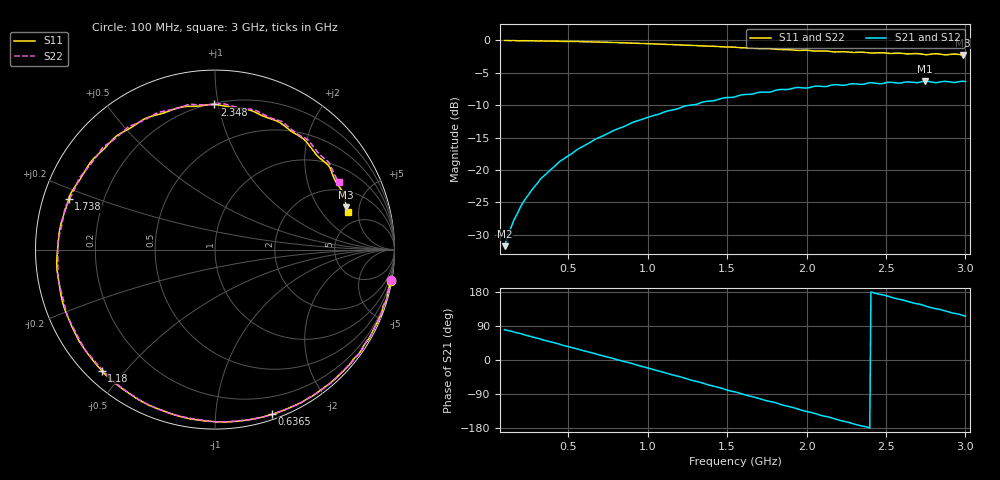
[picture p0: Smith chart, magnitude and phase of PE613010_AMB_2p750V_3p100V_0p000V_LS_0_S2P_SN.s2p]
!Agilent Technologies,N5230A,MY45001685,A.07.50.67
!Agilent N5230A: A.07.50.67
!Date: Monday, March 06, 2017 15:09:25
!Correction: S11(Full 2 Port(1,2))
!S21(Full 2 Port(1,2))
!S12(Full 2 Port(1,2))
!S22(Full 2 Port(1,2))
!S2P File: Measurements: S11, S21, S12, S22:
# Hz S  dB  R 50
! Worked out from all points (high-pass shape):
!   401 points, 100 MHz to 3 GHz, reference 50 ohm
!   highest |S21| = -6.31 dB at 2.746 GHz (marker M1); lowest = -31.7 dB at 100 MHz (marker M2)
!   |S21| within 3 dB of the highest: 1.417 GHz to end of sweep
!   lowest |S11| = -2.3 dB at 2.986 GHz (marker M3), VSWR 7.64, Z = 160 + j184 ohm
!   |S11| at or under -10 dB: nowhere
!   |S22| runs from -2.1 to 0.0 dB; largest |S21 - S12| = 0.0023
!   S11 on the Smith chart (normalised r, x): 100 MHz: 0, -11; 636.5 MHz: 0.04, -1.40; 1.18 GHz: 0.05, -0.43; 1.738 GHz: 0.08, +0.17; 2.348 GHz: 0.21, +0.97; 3 GHz: 3.67, +3.77
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1e8  -0.04 -10.2  -31.74 80.1  -31.77 80.1  -0.03 -9.9
2.015e8  -0.06 -20.9  -25.61 69.5  -25.63 69.5  -0.06 -20.2
2.8125e8  -0.08 -30.3  -22.77 60.0  -22.76 60.1  -0.09 -29.2
4.8425e8  -0.18 -53.7  -18.08 36.9  -18.09 37.0  -0.16 -52.1
5.8575e8  -0.23 -64.7  -16.46 25.6  -16.47 25.6  -0.21 -63.5
6.365e8  -0.25 -70.9  -15.78 20.3  -15.78 20.2  -0.25 -68.0
8.4675e8  -0.40 -94.5  -13.35 -3.3  -13.36 -3.4  -0.37 -91.3
1.0715e9  -0.59 -120.2  -11.38 -29.1  -11.37 -29.2  -0.57 -117.0
1.18025e9  -0.69 -133.1  -10.62 -41.8  -10.62 -41.8  -0.68 -129.3
1.376e9  -0.91 -156.8  -9.40 -64.9  -9.40 -65.0  -0.90 -152.1
1.55e9  -1.08 -176.3  -8.72 -84.1  -8.71 -84.1  -1.05 -170.9
1.7385e9  -1.28 161.0  -8.00 -106.5  -8.00 -106.6  -1.26 166.3
1.898e9  -1.46 142.8  -7.51 -123.5  -7.51 -123.6  -1.42 150.3
1.9705e9  -1.56 134.3  -7.33 -133.0  -7.32 -133.1  -1.49 139.2
2.03575e9  -1.62 127.1  -7.19 -139.0  -7.18 -139.0  -1.56 134.6
2.217e9  -1.77 105.0  -6.92 -160.1  -6.92 -160.2  -1.65 113.2
2.3475e9  -1.85 90.3  -6.80 -174.1  -6.79 -174.1  -1.71 99.7
2.5215e9  -2.04 70.2  -6.48 167.0  -6.46 166.9  -1.92 80.8
2.74625e9  -2.21 44.3  -6.31 142.8  -6.28 142.8  -2.02 57.0
2.80425e9  -2.09 36.9  -6.52 136.1  -6.50 136.2  -1.93 50.3
2.9855e9  -2.29 17.9  -6.33 117.4  -6.32 117.5  -2.11 30.7
3e9  -2.27 15.8  -6.35 115.5  -6.33 115.6  -2.09 28.5
